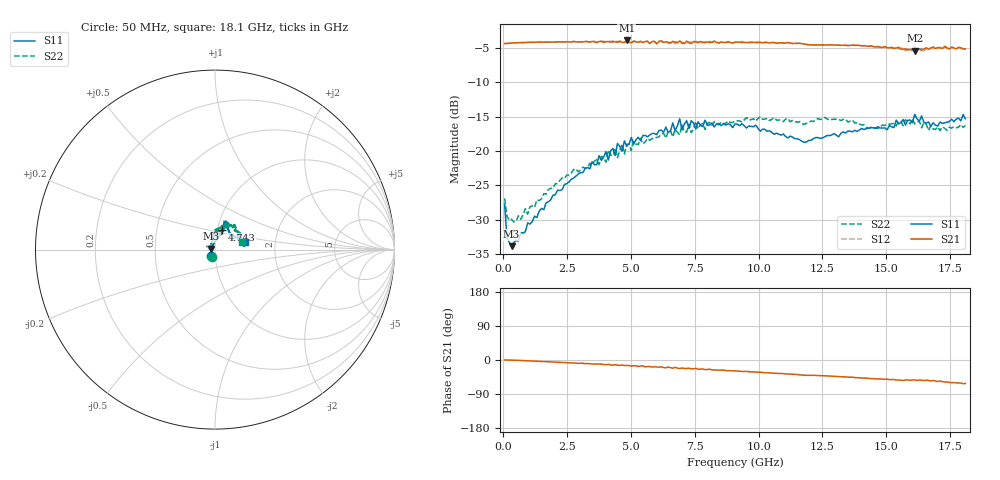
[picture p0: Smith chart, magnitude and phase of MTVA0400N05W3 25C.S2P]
! Network Analyzer HP8720D.06.14 Serial No. US36140669
!  8 Jul 2005  06:21:03
! Frequency  S11  S21  S12  S22
# HZ  S  DB R 50
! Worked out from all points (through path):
!   201 points, 50 MHz to 18.1 GHz, reference 50 ohm
!   highest |S21| = -3.94 dB at 4.833 GHz (marker M1); lowest = -5.4 dB at 16.11 GHz (marker M2)
!   group delay of S21, straight-line fit = 9.61 ps
!   lowest |S11| = -33.8 dB at 320.8 MHz (marker M3), VSWR 1.04, Z = 48.1 + j0.507 ohm
!   |S11| at or under -10 dB: start of sweep to end of sweep
!   |S22| runs from -30.3 to -15.0 dB; largest |S21 - S12| = 0.027
!   S11 on the Smith chart (normalised r, x): 50 MHz: 0.96, -0.07; 4.743 GHz: 1.06, +0.24; 18.1 GHz: 1.39, +0.13
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5e7  -27.73 -120.2  -4.39 0.2  -4.38 0.1  -26.88 -112.5
1.4025e8  -32.46 -156.0  -4.39 -0.0  -4.38 0.1  -29.48 -161.9
3.2075e8  -33.82 165.0  -4.31 -0.2  -4.33 -0.2  -29.91 168.1
3.1185e9  -23.13 77.9  -4.16 -8.6  -4.19 -9.0  -22.35 97.7
4.021e9  -20.08 73.6  -4.11 -12.3  -4.17 -11.4  -21.63 89.2
4.382e9  -20.67 70.8  -4.16 -12.3  -4.14 -13.6  -19.57 88.6
4.47225e9  -18.89 67.1  -4.20 -13.6  -4.07 -12.6  -20.96 91.2
4.65275e9  -20.03 66.9  -4.23 -13.4  -4.06 -14.4  -18.99 89.7
4.743e9  -18.52 69.8  -4.23 -14.5  -4.18 -13.6  -20.43 85.6
4.83325e9  -19.29 74.8  -3.94 -14.4  -4.12 -15.2  -19.05 78.7
6.09675e9  -17.03 67.5  -4.12 -19.1  -4.03 -18.9  -17.95 74.7
6.7285e9  -17.06 72.0  -4.17 -19.4  -4.39 -20.2  -16.89 66.8
6.909e9  -15.32 69.4  -4.01 -22.7  -4.10 -21.1  -17.67 65.7
6.99925e9  -16.94 68.8  -4.26 -21.2  -4.39 -22.9  -16.21 66.4
7.17975e9  -15.60 72.7  -4.04 -22.4  -4.26 -21.3  -17.25 61.3
7.54075e9  -16.82 63.8  -4.17 -22.1  -4.06 -24.6  -15.71 67.8
9.075e9  -16.07 64.4  -4.20 -28.8  -4.17 -28.8  -15.65 54.9
1.21435e10  -18.20 44.8  -4.59 -40.4  -4.53 -40.5  -15.71 53.3
1.512175e10  -16.31 13.8  -5.03 -51.8  -4.85 -51.6  -16.11 41.1
1.61145e10  -14.68 11.6  -5.41 -52.7  -5.07 -53.3  -16.06 32.9
1.674625e10  -16.43 10.3  -5.01 -55.2  -5.19 -55.5  -16.33 25.0
1.81e10  -15.32 14.9  -5.17 -61.9  -5.29 -61.9  -16.29 15.4
